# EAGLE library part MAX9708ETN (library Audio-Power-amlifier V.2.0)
The MAX9708 mono/stereo, Class D audio power amplifier delivers up to 2 x 21W into an 8Ω stereo mode and 1 x 42W into a 4Ω load in mono mode while offering up to 87% efficiency. The MAX9708 provides Class AB amplifier performance with the benefits of Class D efficiency, eliminating the need for a bulky heatsink and conserving power. The MAX9708 operates from a single +10V to +18V supply, driving the load in a BTL configuration. The MAX9708
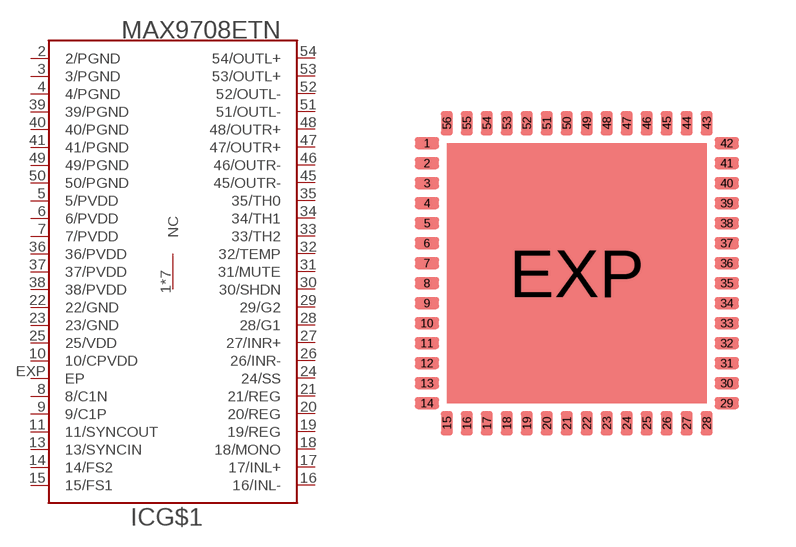
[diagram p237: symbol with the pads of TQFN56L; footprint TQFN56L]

Designator prefix IC; gates G$1=MAX9708ETN G$2=NC

## MAX9708ETN  [TQFN56L]
1  G$2:NC  nc
2  G$1:2/PGND  pwr
3  G$1:3/PGND  pwr
4  G$1:4/PGND  pwr
5  G$1:5/PVDD  pwr
6  G$1:6/PVDD  pwr
7  G$1:7/PVDD  pwr
8  G$1:8/C1N
9  G$1:9/C1P
10  G$1:10/CPVDD  pwr
11  G$1:11/SYNCOUT  out
12  G$2:NC  nc
13  G$1:13/SYNCIN  in
14  G$1:14/FS2
15  G$1:15/FS1
16  G$1:16/INL-  in
17  G$1:17/INL+  in
18  G$1:18/MONO  in
19  G$1:19/REG  out
20  G$1:20/REG  out
21  G$1:21/REG  out
22  G$1:22/GND  pwr
23  G$1:23/GND  pwr
24  G$1:24/SS
25  G$1:25/VDD  pwr
26  G$1:26/INR-  in
27  G$1:27/INR+  in
28  G$1:28/G1  in
29  G$1:29/G2  in
30  G$1:30/SHDN  in
31  G$1:31/MUTE  in
32  G$1:32/TEMP  out
33  G$1:33/TH2  in
34  G$1:34/TH1  in
35  G$1:35/TH0  in
36  G$1:36/PVDD  pwr
37  G$1:37/PVDD  pwr
38  G$1:38/PVDD  pwr
39  G$1:39/PGND  pwr
40  G$1:40/PGND  pwr
41  G$1:41/PGND  pwr
42  G$2:NC  nc
43  G$2:NC  nc
44  G$2:NC  nc
45  G$1:45/OUTR-  out
46  G$1:46/OUTR-  out
47  G$1:47/OUTR+  out
48  G$1:48/OUTR+  out
49  G$1:49/PGND  pwr
50  G$1:50/PGND  pwr
51  G$1:51/OUTL-  out
52  G$1:52/OUTL-  out
53  G$1:53/OUTL+  out
54  G$1:54/OUTL+  out
55  G$2:NC  nc
56  G$2:NC  nc
EXP  G$1:EP  pwr

## Footprint TQFN56L (pad centres in mm)
TQFN56L-8x8x0,8mm www.maxim-ic.com/packages
smd 0.61 x 0.305: 1 -3.75,3.25; 2 -3.75,2.75; 3 -3.75,2.25; 4 -3.75,1.75; 5 -3.75,1.25; 6 -3.75,0.75; 7 -3.75,0.25; 8 -3.75,-0.25; 9 -3.75,-0.75; 10 -3.75,-1.25; 11 -3.75,-1.75; 12 -3.75,-2.25; 13 -3.75,-2.75; 14 -3.75,-3.25; 29 3.75,-3.25; 30 3.75,-2.75; 31 3.75,-2.25; 32 3.75,-1.75; 33 3.75,-1.25; 34 3.75,-0.75; 35 3.75,-0.25; 36 3.75,0.25; 37 3.75,0.75; 38 3.75,1.25; 39 3.75,1.75; 40 3.75,2.25; 41 3.75,2.75; 42 3.75,3.25
smd 0.305 x 0.61: 15 -3.25,-3.75; 16 -2.75,-3.75; 17 -2.25,-3.75; 18 -1.75,-3.75; 19 -1.25,-3.75; 20 -0.75,-3.75; 21 -0.25,-3.75; 22 0.25,-3.75; 23 0.75,-3.75; 24 1.25,-3.75; 25 1.75,-3.75; 26 2.25,-3.75; 27 2.75,-3.75; 28 3.25,-3.75; 43 3.25,3.75; 44 2.75,3.75; 45 2.25,3.75; 46 1.75,3.75; 47 1.25,3.75; 48 0.75,3.75; 49 0.25,3.75; 50 -0.25,3.75; 51 -0.75,3.75; 52 -1.25,3.75; 53 -1.75,3.75; 54 -2.25,3.75; 55 -2.75,3.75; 56 -3.25,3.75
smd 6.5 x 6.5: EXP 0,0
